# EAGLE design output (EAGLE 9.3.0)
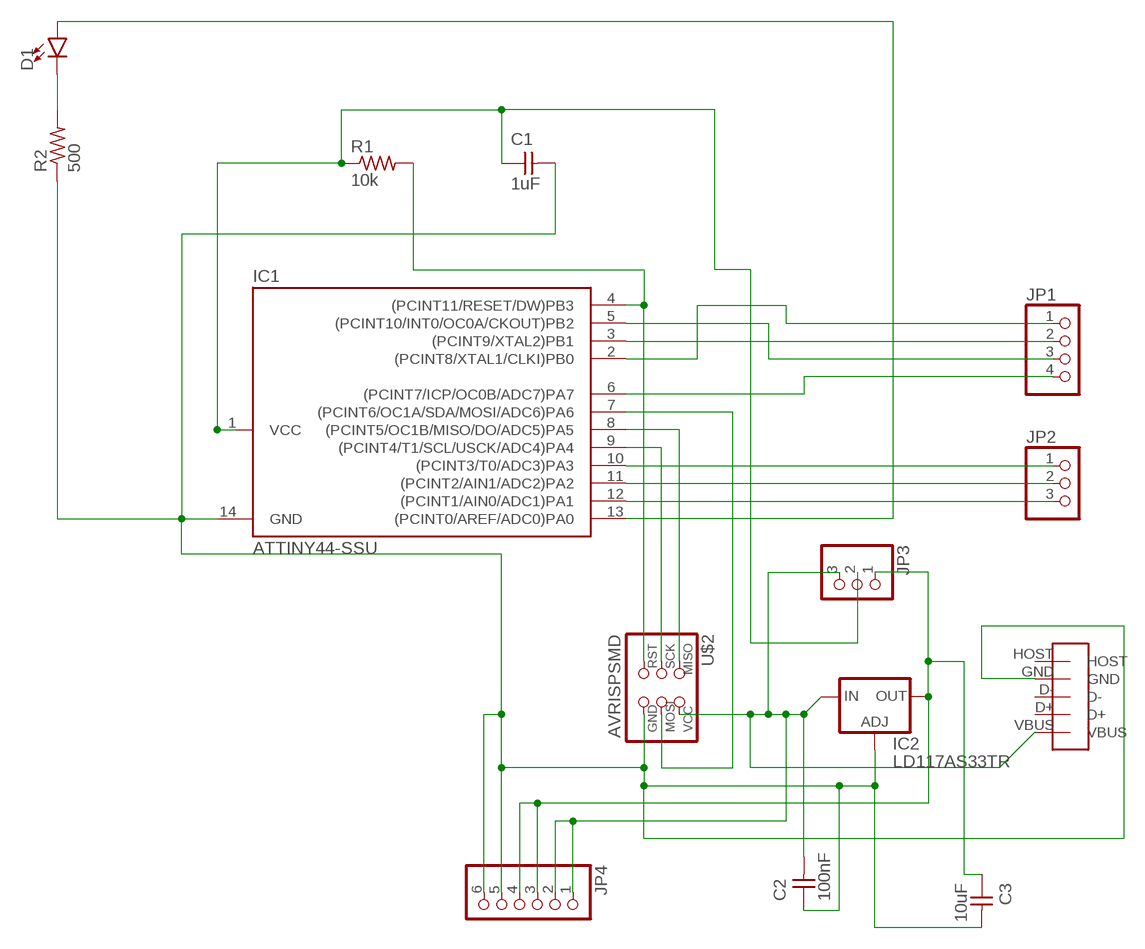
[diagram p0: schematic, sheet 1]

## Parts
C1  1uF  CAP-UNPOLARIZEDFAB  [C1206FAB]
C2  100nF  CAP-UNPOLARIZEDFAB  [C1206FAB]
C3  10uF  CAP-UNPOLARIZEDFAB  [C1206FAB]
D1  LED1206  [LED-1206]
IC1  ATTINY44-SSU  [SOIC14]
IC2  LD117AS33TR  [SOT223]
JP1  PINHD-1X41X04_SMT  [1X04_SMT]
JP2  PINHD-1X31X03_SMT  [1X03_SMT]
JP3  PINHD-1X31X03_SMT  [1X03_SMT]
JP4  PINHD-1X61X06_SMT  [1X06_SMT]
R1  10k  RES-US1206FAB  [R1206FAB]
R2  500  RES-US1206FAB  [R1206FAB]
U$1  MICRO-USB-VERTICAL  [MICRO-USB-VERTICAL]
U$2  AVRISPSMD  [2X03SMD]

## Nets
N$1: C1.1 IC1.1(VCC) JP3.2 R1.1
N$2: IC1.5((PCINT10/INT0/OC0A/CKOUT)PB2) JP1.3
N$3: C3.1 IC2.4(OUT) JP3.1 JP4.3 JP4.4
N$4: IC1.3((PCINT9/XTAL2)PB1) JP1.2
N$5: IC1.8((PCINT5/OC1B/MISO/DO/ADC5)PA5) U$2.1(MISO)
N$6: IC1.9((PCINT4/T1/SCL/USCK/ADC4)PA4) U$2.3(SCK)
N$7: IC1.4((PCINT11/RESET/DW)PB3) R1.2 U$2.5(RST)
N$8: IC1.2((PCINT8/XTAL1/CLKI)PB0) JP1.1
N$9: D1.C R2.2
N$10: IC1.7((PCINT6/OC1A/SDA/MOSI/ADC6)PA6) U$2.4(MOSI)
N$11: D1.A IC1.13((PCINT0/AREF/ADC0)PA0)
N$12: IC1.12((PCINT1/AIN0/ADC1)PA1) JP2.3
N$13: IC1.11((PCINT2/AIN1/ADC2)PA2) JP2.2
N$14: IC1.10((PCINT3/T0/ADC3)PA3) JP2.1
N$15: IC1.6((PCINT7/ICP/OC0B/ADC7)PA7) JP1.4
N$17: C2.2 IC2.3(IN) JP3.3 JP4.1 JP4.2 U$1.VBUS U$2.2(VCC)
N$18: C1.2 C2.1 C3.2 IC1.14(GND) IC2.1(ADJ) JP4.5 JP4.6 R2.1 U$1.GND U$2.6(GND)
Unconnected: U$1.D+ U$1.D- U$1.HOST

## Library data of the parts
C1-C3 = fab:CAP-UNPOLARIZED
D1 = SparkFun-LED:LED: LED (Generic)
IC1 = fab:ATTINY44
IC2 = v-reg:LD117A?*: Low drop fixed and adjustable positive voltage regulators 1 A Source: http://www.st.com/stonline/products/literature/ds/7194/ld1117axx.pdf
JP1 = pinhead+:PINHD-1X4: PIN HEADER
JP2 JP3 = pinhead+:PINHD-1X3: PIN HEADER
JP4 = pinhead+:PINHD-1X6: PIN HEADER
R1 R2 = fab:RES-US: Resistor (US Symbol)
U$1 = custom_micro_usb:MICRO-USB-VERTICAL
U$2 = fab:AVRISP

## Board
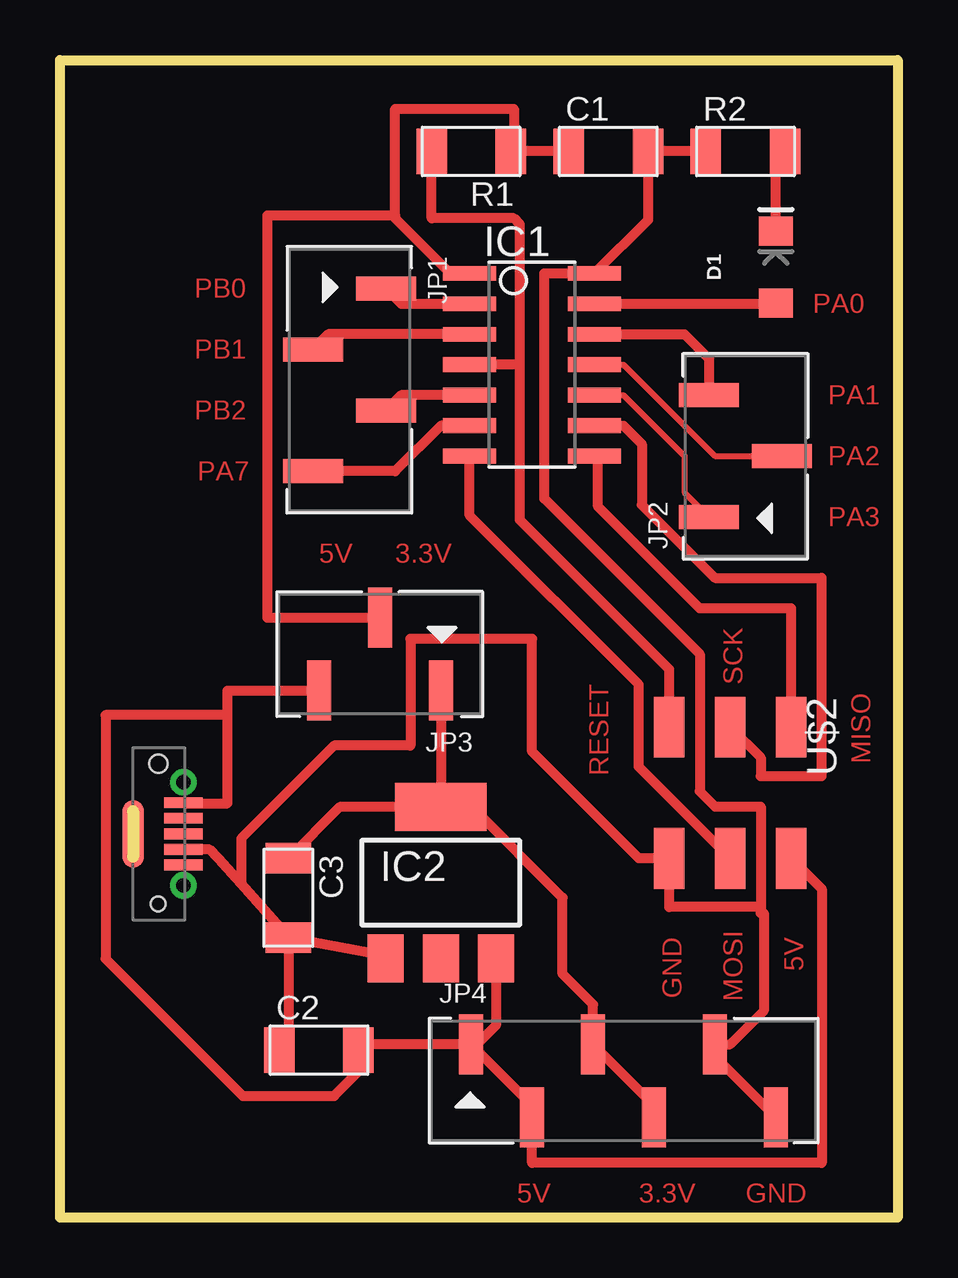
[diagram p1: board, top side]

Size 34.92 x 48.26 mm. Coordinates in mm from the lower left corner, seen from the top.
Outline: 34.92,0 0,0 0,48.26 34.92,48.26 34.92,0
Copper layers (1*16): Top 0.035mm / dielectric 1.5mm / Bottom 0.035mm
Design rules "default": minimum track width 6mil, minimum drill 0.35mm, track to track 6mil, track to pad 6mil, pad to pad 6mil, via to via 6mil, smd to smd 6mil, copper to edge 40mil, drill to drill 6mil, minimum pad ring 10mil, minimum via ring 8mil, stop-mask expansion 4mil, vias tented up to drill 0mil, thermal gap 10mil

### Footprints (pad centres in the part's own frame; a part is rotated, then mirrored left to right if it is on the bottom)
C1206FAB = smd 1.27 x 1.905: 1 -1.651,0; 2 1.651,0
LED-1206 = smd 1.2 x 1.4: A -1.5,0; C 1.5,0
SOIC14 = smd 0.61 x 2.21: 1 -3.81,-2.603; 2 -2.54,-2.603; 3 -1.27,-2.603; 4 0,-2.603; 5 1.27,-2.603; 6 2.54,-2.603; 7 3.81,-2.603; 8 3.81,2.603; 9 2.54,2.603; 10 1.27,2.603; 11 0,2.603; 12 -1.27,2.603; 13 -2.54,2.603; 14 -3.81,2.603
SOT223 = smd 1.5 x 2: 1 -2.3,-3.15; 2 0,-3.15; 3 2.3,-3.15 | smd 3.8 x 2: 4 0,3.15
1X04_SMT = smd 1 x 2.5: 1 -3.81,1.52; 2 -1.27,-1.52; 3 1.27,1.52; 4 3.81,-1.52
1X03_SMT = smd 1 x 2.5: 1 -2.54,1.52; 2 0,-1.52; 3 2.54,1.52
1X06_SMT = smd 1 x 2.5: 1 -6.35,1.52; 2 -3.81,-1.52; 3 -1.27,1.52; 4 1.27,-1.52; 5 3.81,1.52; 6 6.35,-1.52
R1206FAB = smd 1.27 x 1.905: 1 -1.651,0; 2 1.651,0
MICRO-USB-VERTICAL = smd 0.45 x 1.6: D+ -0.65,2.1; D- 0,2.1; GND 0.65,2.1; HOST 1.3,2.1; VBUS -1.3,2.1 | drill 0.6 pad 1.016: S1 -2.15,2.1; S2 2.15,2.1 | smd 2.8 x 0.9: S3 0,0 | hole 0.6: 2.92,1.05 | hole 0.75: -2.92,1.05
2X03SMD = smd 2.54 x 1.27: 1 -2.54,2.54; 2 2.92,2.54; 3 -2.54,0; 4 2.92,0; 5 -2.54,-2.54; 6 2.92,-2.54

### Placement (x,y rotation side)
C1  22.86,44.45 0 top
C2  10.79,6.99 0 top
C3  9.53,13.34 270 top
D1  29.84,39.62 90 top
IC1  19.69,35.56 270 top
IC2  15.87,13.97 0 top
JP1  12.06,34.92 270 top
JP2  28.57,31.75 90 top
JP3  13.33,23.5 180 top
JP4  23.49,5.71 0 top
R1  17.14,44.45 180 top
R2  28.57,44.45 0 top
U$1  3.05,16 270 top
U$2  27.94,17.91 270 top

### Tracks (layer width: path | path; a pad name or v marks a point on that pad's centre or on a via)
N$1
  Top 0.406: C1.1 R1.1 18.92,44.58 18.92,46.23 13.97,46.23 13.97,41.78 | 13.97,41.78 8.64,41.78 8.64,25.02 JP3.2 | IC1.1 16.26,39.37 13.97,41.66 13.97,41.78
N$2
  Top 0.406: IC1.5 14.22,34.29 JP1.3
N$3
  Top 0.152: JP4.4 24.77,4.7 | IC2.4 17.17,17.12
  Top 0.406: JP3.1 IC2.4 11.66,17.12 C3.1 | 24.77,4.7 JP4.3 22.23,8.89 20.95,10.16 20.95,13.34 17.17,17.12
N$4
  Top 0.406: JP1.2 11.18,36.83 IC1.3
N$5
  Top 0.406: IC1.8 22.43,31.61 22.43,29.64 26.67,25.4 30.48,25.4 U$2.1
N$6
  Top 0.406: IC1.9 23.49,33.02 24.26,32.26 24.26,29.72 27.3,26.67 31.75,26.67 31.75,18.41 29.21,18.41 29.21,19.18 U$2.3
N$7
  Top 0.406: 19.18,35.56 IC1.4 | 19.18,35.56 19.18,41.4 18.92,41.66 15.49,41.66 R1.2 | U$2.5 25.4,22.86 19.18,29.08 19.18,35.56
N$8
  Top 0.406: JP1.1 14.22,38.1 IC1.2
N$9
  Top 0.406: D1.C 29.84,44.07 R2.2
N$10
  Top 0.406: IC1.7 17.08,29.27 24.13,22.23 24.13,18.8 U$2.4
N$11
  Top 0.406: D1.A 29.84,38.1 IC1.13
N$12
  Top 0.406: IC1.12 26.03,36.83 27.05,35.81 JP2.3
N$13
  Top 0.254: IC1.11 23.49,35.56 27.3,31.75 JP2.2
N$14
  Top 0.254: IC1.10 23.49,34.29 26.03,31.75 26.03,30.23 JP2.1
N$15
  Top 0.406: IC1.6 15.87,33.02 13.97,31.11 JP1.4
N$17
  Top 0.152: 18.17,10.17 IC2.3 | JP4.2 19.69,4.7 | 17.27,7.11 JP4.1 | U$1.VBUS 5.18,17.27 | 12.7,7.24 C2.2 12.45,6.1
  Top 0.406: 19.69,4.7 17.27,7.11 18.17,8.02 IC2.3 | JP3.3 6.98,21.98 6.98,20.95 | 5.18,17.27 6.98,17.27 6.98,20.95 | JP4.1 12.7,7.24 | 12.45,6.1 11.43,5.08 7.62,5.08 1.9,10.79 1.9,20.95 6.98,20.95 | U$2.2 31.75,13.72 31.75,2.29 19.69,2.29 JP4.2
N$18
  Top 0.152: JP4.5 27.3,6.74 | 13.08,10.33 IC2.1 | 13.57,10.94 IC2.1 | IC2.1 13.97,11.21 | 9.53,7.37 C2.1
  Top 0.406: R2.1 C1.2 24.51,41.59 IC1.14 20.19,39.37 20.19,29.97 26.67,23.5 26.67,17.78 27.3,17.14 29.21,17.14 29.21,12.95 | 29.21,12.95 29.21,12.7 29.34,12.7 29.34,8.63 27.94,7.24 JP4.5 | 29.21,12.95 25.4,12.95 U$2.6 24.13,14.99 19.69,19.43 19.69,24.13 14.6,24.13 14.6,19.69 11.43,19.69 7.55,15.81 7.55,13.91 | 27.3,6.74 JP4.6 | C3.2 13.57,10.94 | C3.2 7.55,13.91 | 7.55,13.91 6.6,14.99 6.24,15.35 U$1.GND | C3.2 9.53,7.37

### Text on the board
Top: PB0 | PA0 | PB1 | PA1 | PB2 | PA7 | PA2 | PA3 | 5V | 3.3V | SCK | MISO | RESET | 5V | GND | MOSI | 5V | 3.3V | GND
